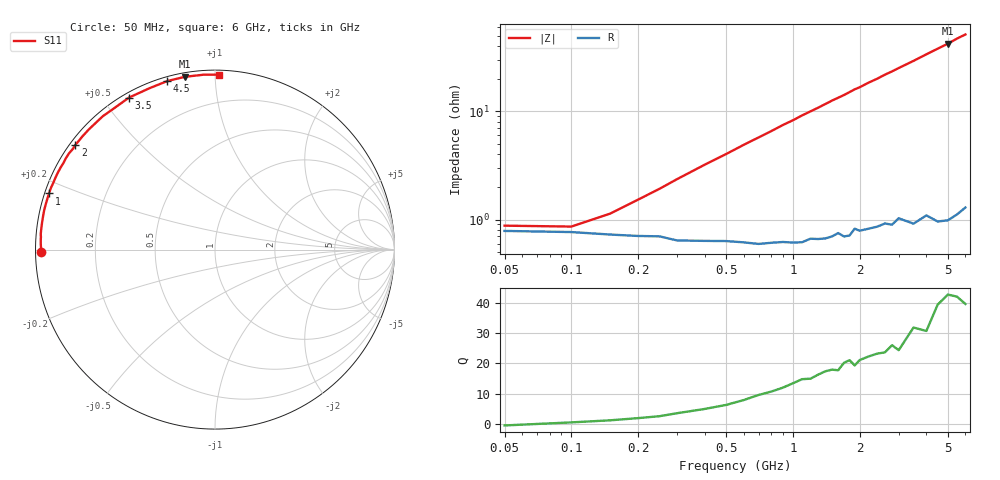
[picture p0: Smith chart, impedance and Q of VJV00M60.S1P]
! Infineon Technologies  Discrete & RF Semiconductors
! BB 914
! Si Tuning Diode in SOT23
! VR =
! S-Parameters:  July  1999
# GHz  S  MA  R  50
!  f  S11
! GHz  MAG  ANG
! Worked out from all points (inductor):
!   34 points, 50 MHz to 6 GHz, reference 50 ohm
!   read as one part to ground: L = 1.25 nH near 300 MHz
!   highest Q = 42.1 at 5 GHz (marker M1), where L = 1.34 nH
!   S11 on the Smith chart (normalised r, x): 50 MHz: 0.02, -0.01; 1 GHz: 0.01, +0.16; 2 GHz: 0.02, +0.33; 3.5 GHz: 0.02, +0.58; 4.5 GHz: 0.02, +0.76; 6 GHz: 0.03, +1.02
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0.05  0.9691 -179.1
0.1  0.9698 179.1
0.3  0.9748 174.8
0.4  0.975 172.8
0.6  0.9759 168.9
0.7  0.9768 167.0
0.8  0.9763 165.1
0.9  0.976 163.1
1  0.9764 161.3
1.1  0.9764 159.3
1.3  0.9751 155.7
1.5  0.9741 151.9
1.6  0.9724 150.2
1.7  0.9745 148.5
1.8  0.9742 146.6
1.9  0.9706 144.7
2  0.972 143.2
2.2  0.9714 139.6
2.4  0.9708 136.5
2.6  0.9696 133.0
2.8  0.971 130.0
3  0.9677 126.8
3.5  0.973 119.5
4  0.9703 112.3
4.5  0.9759 105.8
5  0.9772 99.9
5.5  0.9766 93.7
6  0.9751 88.7
